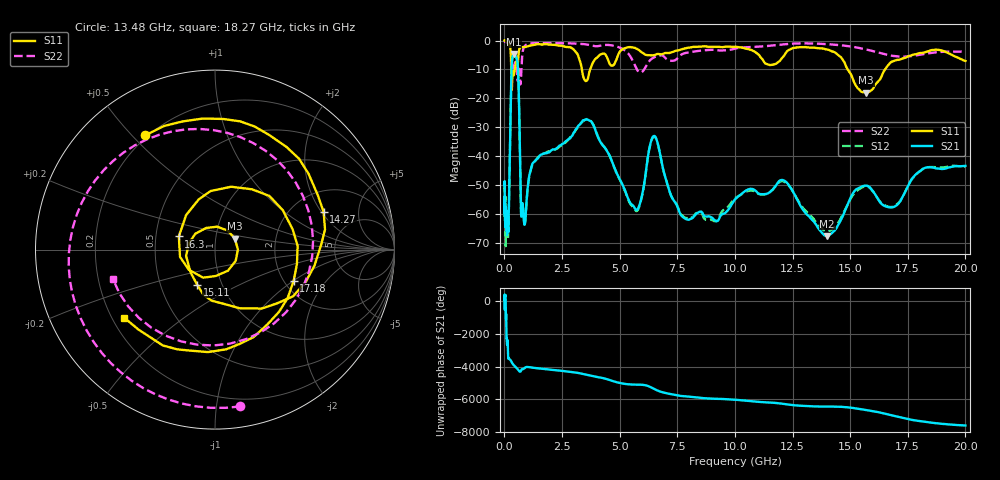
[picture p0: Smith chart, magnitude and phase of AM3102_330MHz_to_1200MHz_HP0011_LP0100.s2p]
! Date/Time: Tue, Sep 11, 2018 5:11 PM
! Network Analyzer: Agilent Technologies E8362B Rev: A.07.50.63
! Sweep from 0.010 to 20.000 GHz, 1601 Points, Sweep Type: LOG
! Power Supply: 4.950 V, 0.001 A
# Hz S DB R 50
!freq MagS11 AngS11 MagS21 AngS21 MagS12 AngS12 MagS22 AngS22
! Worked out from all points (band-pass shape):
!   1601 points, 10 MHz to 20 GHz, reference 50 ohm
!   highest |S21| = -4.60 dB at 414.5 MHz (marker M1); lowest = -67.6 dB at 14.01 GHz (marker M2)
!   |S21| within 3 dB of the highest: 325.6 MHz to 570.8 MHz (245.2 MHz wide, 54.7 % of centre)
!   lowest |S11| = -18.0 dB at 15.7 GHz (marker M3), VSWR 1.29, Z = 61.9 + j7.65 ohm
!   |S11| at or under -10 dB: 298.6 MHz to 449.5 MHz (150.9 MHz wide, 40.3 % of centre); 3.362 GHz to 3.722 GHz (360.7 MHz wide, 10.2 % of centre); 14.89 GHz to 16.51 GHz (1.62 GHz wide, 10.3 % of centre)
!   |S22| runs from -15.2 to -0.2 dB; largest |S21 - S12| = 0.0095
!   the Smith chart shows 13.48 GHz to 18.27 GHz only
!   S11 on the Smith chart (normalised r, x): 13.48 GHz: 0.19, +0.55; 14.27 GHz: 2.94, +2.10; 15.11 GHz: 0.76, -0.31; 16.3 GHz: 0.66, +0.10; 17.18 GHz: 2.25, -1.01; 18.27 GHz: 0.25, -0.32
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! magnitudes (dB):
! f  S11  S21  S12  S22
! 10 MHz  0.0  -50.0  -49.8  -0.2
! 35.55 MHz  0.0  -64.0  -60.5  -0.4
! 126.4 MHz  -0.4  -63.1  -67.0  -0.8
! 186.6 MHz  -1.0  -62.0  -62.0  -1.2
! 414.5 MHz  -11.9  -4.6  -4.7  -9.1
! 447.2 MHz  -10.1  -4.8  -4.8  -7.9
! 594.7 MHz  -6.8  -10.6  -10.7  -13.1
! 736.5 MHz  -2.2  -60.9  -61.1  -9.6
! 1.59 GHz  -1.4  -39.4  -39.5  -0.9
! 3.668 GHz  -11.5  -27.6  -27.2  -1.5
! 5.652 GHz  -2.5  -57.9  -58.3  -8.4
! 6.487 GHz  -5.1  -33.0  -33.2  -5.8
! 7.845 GHz  -2.7  -61.6  -61.3  -4.3
! 13.48 GHz  -2.5  -63.2  -62.4  -1.1
! 14.01 GHz  -3.1  -67.6  -65.9  -1.3
! 14.27 GHz  -3.9  -66.1  -64.9  -1.4
! 15.11 GHz  -13.2  -53.0  -53.5  -2.2
! 15.7 GHz  -18.0  -50.2  -50.5  -3.1
! 16.3 GHz  -13.4  -56.0  -55.8  -4.3
! 17.18 GHz  -6.5  -55.5  -55.4  -5.6
! 18.27 GHz  -4.0  -43.9  -44.0  -4.5
! 20 GHz  -7.1  -43.3  -43.7  -3.8
